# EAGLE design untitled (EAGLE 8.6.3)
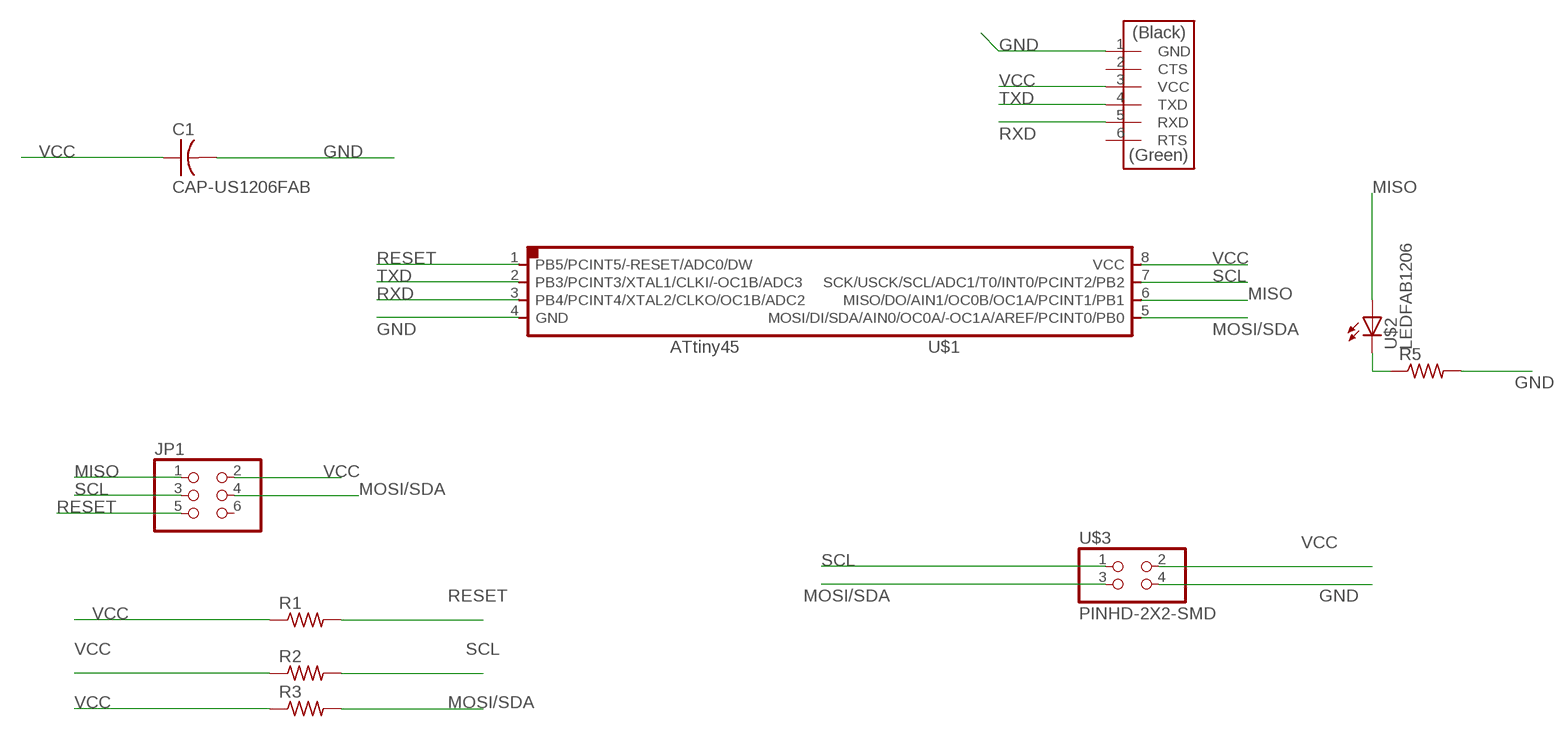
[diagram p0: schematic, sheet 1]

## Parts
C1  CAP-US1206FAB  [C1206FAB]
JP1  PINHD-2X3-SMD  [2X03SMD]
R1  RES-US1206FAB  [R1206FAB]
R2  RES-US1206FAB  [R1206FAB]
R3  RES-US1206FAB  [R1206FAB]
R5  RES-US1206FAB  [R1206FAB]
U$1  ATTINY45SI  [SOIC8]
U$2  LEDFAB1206  [LED1206FAB]
U$3  PINHD-2X2-SMD  [2X02SMD]
U$4  FTDI-SMD-HEADER  [1X06SMD]

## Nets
GND: C1.2 R5.2 U$1.4(GND) U$3.4 U$4.1(GND)
MISO: JP1.1 U$1.6(MISO/DO/AIN1/OC0B/OC1A/PCINT1/PB1) U$2.1(A)
MOSI/SDA: JP1.4 R3.2 U$1.5(MOSI/DI/SDA/AIN0/OC0A/-OC1A/AREF/PCINT0/PB0) U$3.3
N$1: R5.1 U$2.2(C)
RESET: JP1.5 R1.2 U$1.1(PB5/PCINT5/-RESET/ADC0/DW)
RXD: U$1.3(PB4/PCINT4/XTAL2/CLKO/OC1B/ADC2) U$4.5(RXD)
SCL: JP1.3 R2.2 U$1.7(SCK/USCK/SCL/ADC1/T0/INT0/PCINT2/PB2) U$3.1
TXD: U$1.2(PB3/PCINT3/XTAL1/CLKI/-OC1B/ADC3) U$4.4(TXD)
VCC: C1.1 JP1.2 R1.1 R2.1 R3.1 U$1.8(VCC) U$3.2 U$4.3(VCC)
Unconnected: JP1.6 U$4.2(CTS) U$4.6(RTS)

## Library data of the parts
C1 = fab:CAP-US
JP1 = fab:PINHD-2X3-SMD: PIN HEADER
R1-R3 R5 = fab:RES-US: Resistor (US Symbol)
U$1 = fab:ATTINY45
U$2 = fab:LED: LED
U$3 = fab:PINHD-2X2-SMD
U$4 = fab:FTDI-SMD-HEADER

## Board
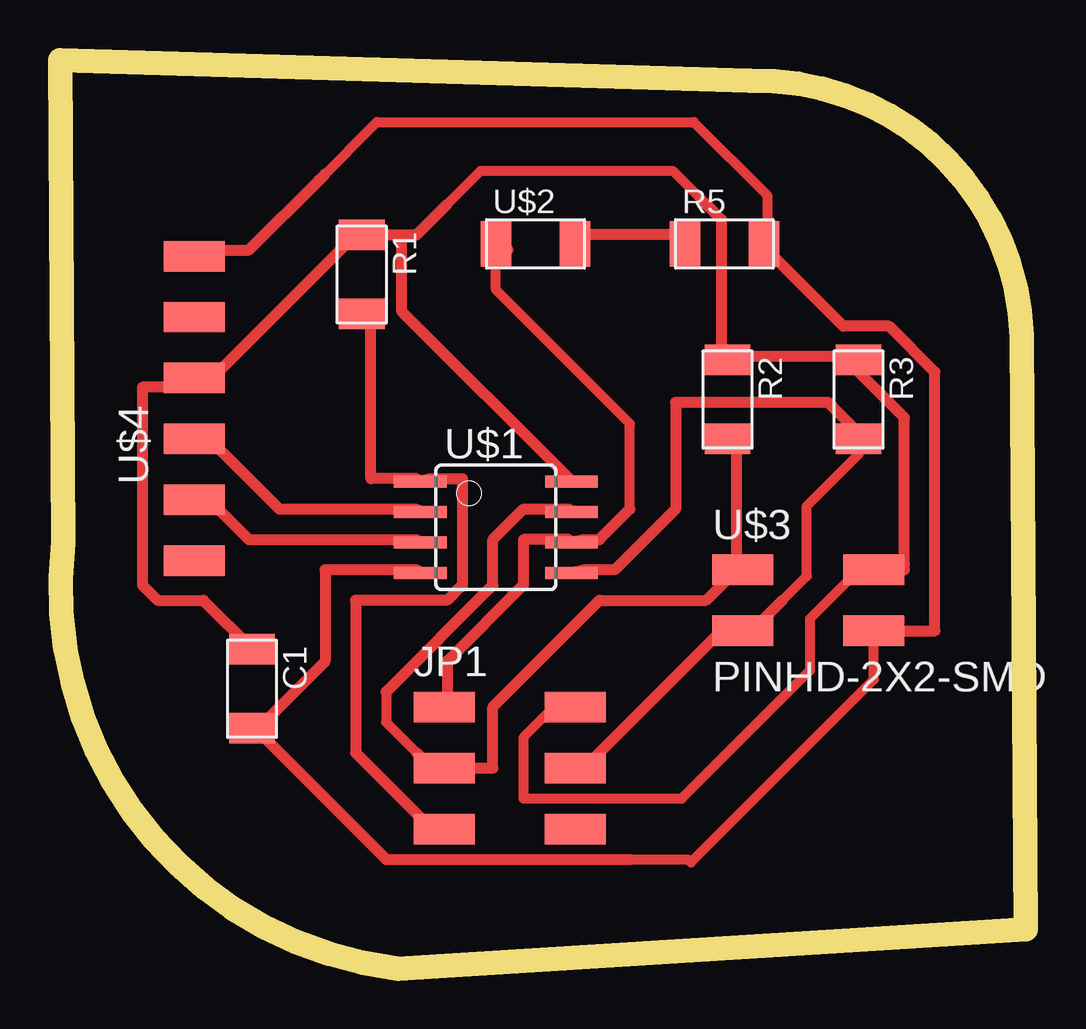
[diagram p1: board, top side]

Size 40.24 x 37.89 mm. Coordinates in mm from the lower left corner, seen from the top.
Outline: 0,37.89 0.14,17.77 arc90 14.1,0 40.24,1.64 40.07,26.38 arc90 28.73,37.02 0,37.89
Copper layers (1*16): Top 0.035mm / dielectric 1.5mm / Bottom 0.035mm
Design rules "default *": minimum track width 18mil, minimum drill 0.35mm, track to track 16mil, track to pad 16mil, pad to pad 16mil, via to via 16mil, smd to smd 16mil, copper to edge 40mil, drill to drill 6mil, minimum pad ring 10mil, minimum via ring 8mil, stop-mask expansion 4mil, vias tented up to drill 0mil, thermal gap 10mil

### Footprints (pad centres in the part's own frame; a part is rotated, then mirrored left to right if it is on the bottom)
C1206FAB = smd 1.27 x 1.905: 1 -1.651,0; 2 1.651,0
2X03SMD = smd 2.54 x 1.27: 1 -2.54,2.54; 2 2.92,2.54; 3 -2.54,0; 4 2.92,0; 5 -2.54,-2.54; 6 2.92,-2.54
R1206FAB = smd 1.27 x 1.905: 1 -1.651,0; 2 1.651,0
SOIC8 = smd 0.5 x 2.2: 1 -1.905,-3.154; 2 -0.645,-3.154; 3 0.625,-3.154; 4 1.895,-3.154; 5 1.905,3.154; 6 0.635,3.154; 7 -0.635,3.154; 8 -1.905,3.154
LED1206FAB = smd 1.27 x 1.905: 1 -1.651,0; 2 1.651,0
2X02SMD = smd 2.54 x 1.27: 1 -2.54,1.27; 2 2.92,1.27; 3 -2.54,-1.27; 4 2.92,-1.27
1X06SMD = smd 2.54 x 1.27: 1 0,6.35; 2 0,3.81; 3 0,1.27; 4 0,-1.27; 5 0,-3.81; 6 0,-6.35

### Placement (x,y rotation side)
C1  8,11.67 270 top
JP1  18.54,8.37 0 top
R1  12.57,28.95 270 top
R2  27.81,23.74 270 top
R3  33.27,23.74 270 top
R5  27.69,30.22 0 top
U$1  18.16,18.41 270 top
U$2  19.81,30.22 0 top
U$3  30.99,15.36 0 top
U$4  5.59,23.36 0 top

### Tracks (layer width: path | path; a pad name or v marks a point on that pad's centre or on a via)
GND
  Top 0.406: 10.79,32.88 13.21,35.3 26.42,35.3 29.46,32.25 29.46,29.96 29.08,30.34 | 23.75,4.56 26.16,4.56 26.29,4.44 33.91,12.05 U$3.4
  Top 0.457: 11.05,33.14 10.79,32.88 7.87,29.96 5.97,29.96 U$4.1 | U$1.4 14.86,16.63 11.05,16.63 11.05,12.82 8.51,10.28 C1.2 8.51,9.64 13.59,4.56 23.75,4.56 | 33.27,14.09 U$3.4 36.45,14.09 36.45,24.88 34.54,26.79 32.64,26.79 29.65,29.77 29.46,29.96 R5.2
MISO
  Top 0.406: 23.75,19.17 23.75,22.72 18.16,28.31 U$2.1
  Top 0.457: 23.75,19.17 22.48,17.9 21.84,17.9 U$1.6 21.21,17.9 19.3,17.9 19.3,15.99 16.13,12.82 16.13,10.91 JP1.1 | 18.67,29.96 U$2.1
MOSI/SDA
  Top 0.406: 29.65,14.91 31.11,16.37 31.11,19.29 33.27,21.45 33.27,22.34
  Top 0.457: 30.1,15.36 29.65,14.91 28.83,14.09 U$3.3 27.56,14.09 21.84,8.37 JP1.4 | U$1.5 21.84,16.63 23.11,16.63 25.65,19.17 25.65,23.61 32,23.61 33.27,22.34 R3.2
N$1
  Top 0.457: U$2.2 21.84,30.6 25.65,30.6 R5.1
RESET
  Top 0.457: R1.2 12.95,26.79 12.95,20.44 14.86,20.44 U$1.1 15.49,20.44 16.76,20.44 16.76,15.99 16.13,15.36 12.32,15.36 12.32,9.01 15.49,5.83 JP1.5
RXD
  Top 0.457: U$1.3 14.86,17.9 7.87,17.9 6.6,19.17 5.97,19.17 U$4.5
SCL
  Top 0.406: 13.59,11.55 13.59,10.28 14.86,9.01
  Top 0.457: 28.19,16.63 28.19,21.71 R2.2 | 13.59,11.55 18.03,15.99 18.03,17.9 19.3,19.17 21.21,19.17 U$1.7 | 14.86,9.01 15.49,8.37 JP1.3 18.03,8.37 18.03,10.91 22.48,15.36 26.92,15.36 28.19,16.63 | 28.19,16.63 U$3.1
TXD
  Top 0.457: U$1.2 14.86,19.17 9.14,19.17 6.6,21.71 5.97,21.71 U$4.4
VCC
  Top 0.406: 34.67,16.63 33.27,16.63 31.24,14.6 31.24,12.44 25.91,7.1 24.89,7.1 24.38,7.1 19.3,7.1 19.3,9.64 20.57,10.91 21.21,10.91 | 33.53,16.88 35.18,16.88 | 16.13,31.87 17.53,33.26 25.53,33.26 26.92,31.87 | JP1.2 21.59,10.79 21.97,10.79 21.84,10.91 JP1.2
  Top 0.457: 21.21,10.91 JP1.2 | 33.27,16.63 U$3.2 34.67,16.63 35.18,16.63 35.18,16.88 35.18,22.98 33.27,24.88 R3.1 33.27,25.52 28.19,25.52 R2.1 27.56,25.52 27.56,31.23 26.92,31.87 | C1.1 5.97,15.36 4.06,15.36 3.43,15.99 3.43,24.25 5.33,24.25 U$4.3 5.97,24.88 6.6,24.88 12.32,30.6 R1.1 14.22,30.6 | 14.22,30.6 14.22,27.42 21.21,20.44 U$1.8 | 16.13,31.87 14.86,30.6 14.22,30.6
